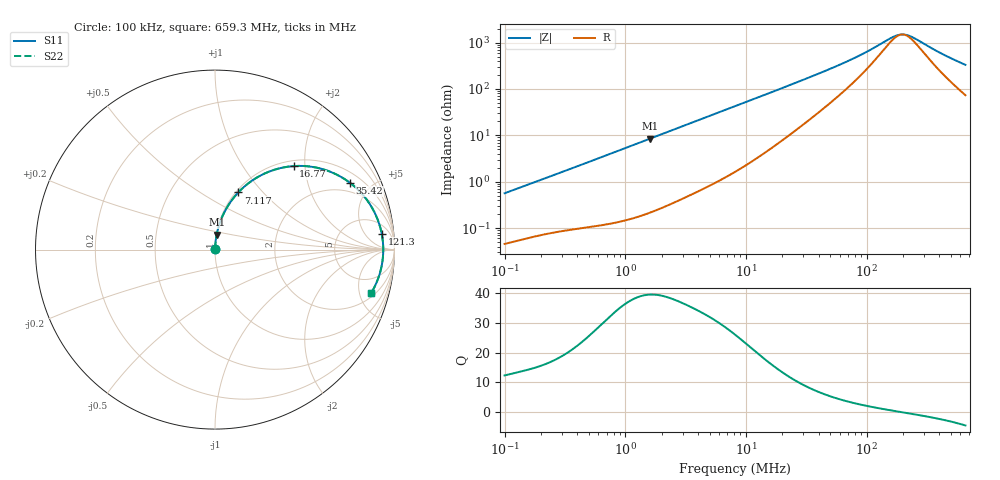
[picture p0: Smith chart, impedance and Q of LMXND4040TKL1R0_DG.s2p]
! LMXND4040TKL1R0_DG  S-PARAMETER MODEL  ( General Type )
! Model Generated by TAIYO YUDEN Corporation (https://www.yuden.co.jp/en/)
! Version 1.0
! TAIYO YUDEN Control No. 191023NI43SB-FBB
! Copyright(c) 2019 TAIYO YUDEN CO.,LTD. All Rights Reserved.
! Product Description (link to TY-COMPAS)
! https://ds.yuden.co.jp/TYCOMPAS/or/detail?pn=LMXND4040TKL1R0NDG&u=M
! Products Name : Inductors
! Characteristics :
!  Inductance : 1.0 uH , SRF(min) : 90 MHz , DC Resistance(max) : 0.0324 Ohm
!  Rated Current : Saturation :4000 mA , Temp Rise : 3200 mA (40 degC)
!  Case Size : 4.0 x 4.0 / 0.157 x 0.157 [mm/inch] , Thickness : 1.8 / 0.071 [mm/inch]
!  (Conditions: Temperature = 25 degC , DC Bias Current/Voltage = 0A / 0V)
! External Node Assignments :
!  1  o---GGG---o  2
! GND o---------o GND
! Frequency Range : 0.1MHz  -  659.336432MHz  [ 402 STEP ]
# MHz S RI R 50
! Freq[MHz].  S11 Real  S11 Imag  S21 Real  S21 Imag  S12 Real  S12 Imag  S22 Real  S22 Imag
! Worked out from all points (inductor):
!   401 points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, 100 kHz to 659.3 MHz, reference 50 ohm
!   read as one part in series: L = 886 nH near 104.5 kHz
!   highest Q = 39.4 at 1.596 MHz (marker M1), where L = 841 nH
!   self-resonance near 198.3 MHz
!   S11 on the Smith chart (normalised r, x): 100 kHz: 1.00, +0.01; 7.117 MHz: 1.03, +0.74; 16.77 MHz: 1.11, +1.75; 35.42 MHz: 1.48, +3.74; 121.3 MHz: 10, +14; 659.3 MHz: 2.47, -6.47
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0.1  0.000486 0.00561  0.9995 -0.00561  0.9995 -0.00561  0.000486 0.00561
0.436215  0.00154 0.0233  0.9985 -0.0233  0.9985 -0.0233  0.00154 0.0233
1.595948  0.00916 0.0834  0.9908 -0.0834  0.9908 -0.0834  0.00916 0.0834
1.902834  0.0125 0.0989  0.9875 -0.0989  0.9875 -0.0989  0.0125 0.0989
4.107454  0.0497 0.2031  0.9503 -0.2031  0.9503 -0.2031  0.0497 0.2031
7.116508  0.1297 0.3185  0.8703 -0.3185  0.8703 -0.3185  0.1297 0.3185
8.300444  0.1671 0.3541  0.8329 -0.3541  0.8329 -0.3541  0.1671 0.3541
11.54298  0.2751 0.4233  0.7249 -0.4233  0.7249 -0.4233  0.2751 0.4233
16.77374  0.4379 0.4652  0.5621 -0.4652  0.5621 -0.4652  0.4379 0.4652
23.84483  0.6016 0.4477  0.3984 -0.4477  0.3984 -0.4477  0.6016 0.4477
35.42044  0.7532 0.3713  0.2468 -0.3713  0.2468 -0.3713  0.7532 0.3713
46.1134  0.8238 0.305  0.1762 -0.305  0.1762 -0.305  0.8238 0.305
61.36888  0.8751 0.2328  0.1249 -0.2328  0.1249 -0.2328  0.8751 0.2328
87.23936  0.9119 0.1523  0.0881 -0.1523  0.0881 -0.1523  0.9119 0.1523
121.319  0.9293 0.0866  0.0707 -0.0866  0.0707 -0.0866  0.9293 0.0866
154.5092  0.9355 0.043  0.0645 -0.043  0.0645 -0.043  0.9355 0.043
172.4619  0.9368 0.0239  0.0632 -0.0239  0.0632 -0.0239  0.9368 0.0239
188.3147  0.9374 0.00883  0.0626 -0.00883  0.0626 -0.00883  0.9374 0.00883
205.6248  0.9374 -0.00619  0.0626 0.00619  0.0626 0.00619  0.9374 -0.00619
224.5259  0.937 -0.0213  0.063 0.0213  0.063 0.0213  0.937 -0.0213
424.7679  0.9161 -0.1398  0.0839 0.1398  0.0839 0.1398  0.9161 -0.1398
659.3364  0.8713 -0.2401  0.1287 0.2401  0.1287 0.2401  0.8713 -0.2401
